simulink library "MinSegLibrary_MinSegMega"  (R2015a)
settings: Solver=ode45  StartTime=0.0  StopTime=10.0  RelTol=1e-3
undefined symbols (not defined in the file or in its folder): PWMoffset, Vsupply
libraries: MinSegLibrary_MinSegMega x7, MinSegLibrary_M1V4 x1

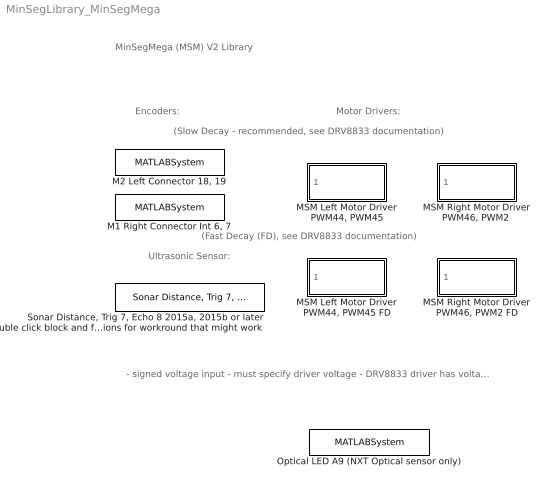
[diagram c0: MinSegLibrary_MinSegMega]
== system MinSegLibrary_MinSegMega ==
  note: (Slow Decay - recommended, see DRV8833 documentation)
  note: Motor Drivers:
  note: Ultrasonic Sensor:
  note: Encoders:
  note: MinSegMega (MSM) V2 Library
  note: (Fast Decay (FD), see DRV8833 documentation)
  note: - signed voltage input - must specify driver voltage - DRV8833 driver has voltage drop of about 0.6 volts, so max usable USB voltage is about 3.9 volts - Fast decay is nonlinear PWM to voltage for NXT motor - look at generic driver block in RASPlib for table lookup and other options
  "M1 Right Connector Int 6, 7" : MATLABSystem  System=Encoder_arduino  Encoder=2  PinA=6  PinB=7  PWMFSelect=3  PWMTimer=-1
  "M2 Left Connector 18, 19" : MATLABSystem  System=Encoder_arduino  Encoder=1  PinA=19  PinB=18  PWMFSelect=3  PWMTimer=-1
  "MSM Left Motor Driver PWM44, PWM45" : Subsystem
  "MSM Left Motor Driver PWM44, PWM45 FD" : Subsystem
  "MSM Right Motor Driver PWM46, PWM2 " : Subsystem
  "MSM Right Motor Driver PWM46, PWM2 FD" : Subsystem
  Optical LED A9 (NXT Optical sensor only) : MATLABSystem  System=soDAnalogWrite  Pin=9
  "Sonar Distance, Trig 7, Echo 8 2015a, 2015b or later double click block and follow instructions for workround that might work" : MinSegLibrary_M1V4/Sonar Distance, Trig 7, Echo 8 2015a, 2015b or later double click block and follow instructions for workround that might work  TrigPin=7  EchoPin=8

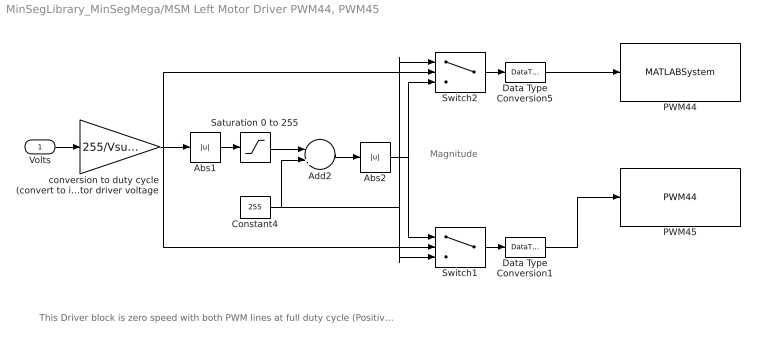
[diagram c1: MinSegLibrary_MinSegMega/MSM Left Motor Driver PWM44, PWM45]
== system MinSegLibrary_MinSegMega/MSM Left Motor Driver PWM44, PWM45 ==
  note: Magnitude
  note: This Driver block is zero speed with both PWM lines at full duty cycle (Positive voltage on both motor terminals). This method produces a linear motor response for DRV8833 driver in both directions and eliminates the typical dead zone when the motor starts. The driver may draw more current in this configuration (has not been verified) The SN754410 driver this has no effect, so the driver could alternatively be modified so that zero speed is zero voltage to both PWM lines.
  Volts : Inport
  Abs1 : Abs
  Abs2 : Abs
  Add2 : Sum  Inputs=-+
  Constant4 : Constant  Value=255
  Data Type Conversion1 : DataTypeConversion  OutDataTypeStr=uint8
  Data Type Conversion5 : DataTypeConversion  OutDataTypeStr=uint8
  PWM44 : MATLABSystem  System=soPWMWrite  Pin=44
  PWM45 : MinSegLibrary_MinSegMega/MSM Left Motor Driver PWM44, PWM45/PWM44  Pin=45
  Saturation 0 to 255 : Saturate  UpperLimit=255  LowerLimit=0
  Switch1 : Switch
  Switch2 : Switch
  conversion to duty cycle (convert to int) denominator is motor driver voltage : Gain  Gain=255/Vsupply  OutDataTypeStr=int16
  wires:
  Data Type Conversion1/1 -> PWM45/1
  Data Type Conversion5/1 -> PWM44/1
  Switch1/1 -> Data Type Conversion1/1
  Switch2/1 -> Data Type Conversion5/1
  Abs2/1 -> Switch1/1, Switch2/3
  Add2/1 -> Abs2/1
  Constant4/1 -> Add2/2, Switch2/1, Switch1/3
  Abs1/1 -> Saturation 0 to 255/1
  Saturation 0 to 255/1 -> Add2/1
  conversion to duty cycle (convert to int) denominator is motor driver voltage/1 -> Switch1/2, Abs1/1, Switch2/2
  Volts/1 -> conversion to duty cycle (convert to int) denominator is motor driver voltage/1

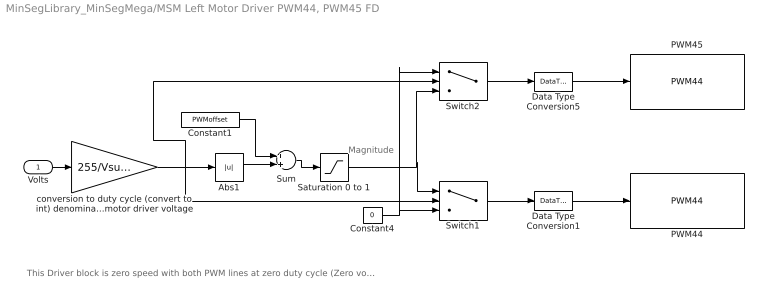
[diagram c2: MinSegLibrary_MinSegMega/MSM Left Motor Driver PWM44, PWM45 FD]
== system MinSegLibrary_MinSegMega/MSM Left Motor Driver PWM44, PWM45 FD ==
  note: Magnitude
  note: This Driver block is zero speed with both PWM lines at zero duty cycle (Zero voltage on both motor terminals). This method produces a nonlinear motor response for DRV8833 driver in both directions and eliminates
  Volts : Inport
  Abs1 : Abs
  Constant1 : Constant  Value=PWMoffset
  Constant4 : Constant  Value=0
  Data Type Conversion1 : DataTypeConversion  OutDataTypeStr=uint8
  Data Type Conversion5 : DataTypeConversion  OutDataTypeStr=uint8
  PWM44 : MinSegLibrary_MinSegMega/MSM Left Motor Driver PWM44, PWM45/PWM44  Pin=44
  PWM45 : MinSegLibrary_MinSegMega/MSM Left Motor Driver PWM44, PWM45/PWM44  Pin=45
  Saturation 0 to 1 : Saturate  UpperLimit=255  LowerLimit=0
  Sum : Sum
  Switch1 : Switch
  Switch2 : Switch
  conversion to duty cycle (convert to int) denominator is motor driver voltage : Gain  Gain=255/Vsupply  OutDataTypeStr=int16
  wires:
  Constant1/1 -> Sum/1
  Sum/1 -> Saturation 0 to 1/1
  Abs1/1 -> Sum/2
  Data Type Conversion1/1 -> PWM44/1
  Data Type Conversion5/1 -> PWM45/1
  Switch1/1 -> Data Type Conversion1/1
  Switch2/1 -> Data Type Conversion5/1
  Saturation 0 to 1/1 -> Switch1/1, Switch2/3
  Constant4/1 -> Switch1/3, Switch2/1
  conversion to duty cycle (convert to int) denominator is motor driver voltage/1 -> Switch2/2, Abs1/1, Switch1/2
  Volts/1 -> conversion to duty cycle (convert to int) denominator is motor driver voltage/1

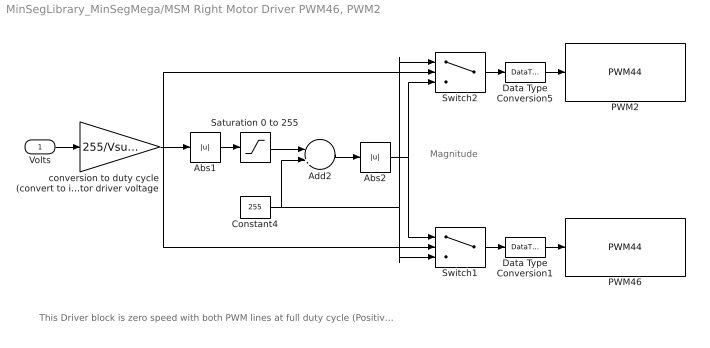
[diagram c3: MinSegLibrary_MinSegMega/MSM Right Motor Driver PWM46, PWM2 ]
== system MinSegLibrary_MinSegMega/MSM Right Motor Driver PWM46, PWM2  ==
  note: Magnitude
  note: This Driver block is zero speed with both PWM lines at full duty cycle (Positive voltage on both motor terminals). This method produces a linear motor response for DRV8833 driver in both directions and eliminates the typical dead zone when the motor starts. The driver may draw more current in this configuration (has not been verified) The SN754410 driver this has no effect, so the driver could alternatively be modified so that zero speed is zero voltage to both PWM lines.
  Volts : Inport
  Abs1 : Abs
  Abs2 : Abs
  Add2 : Sum  Inputs=-+
  Constant4 : Constant  Value=255
  Data Type Conversion1 : DataTypeConversion  OutDataTypeStr=uint8
  Data Type Conversion5 : DataTypeConversion  OutDataTypeStr=uint8
  PWM2 : MinSegLibrary_MinSegMega/MSM Left Motor Driver PWM44, PWM45/PWM44  Pin=2
  PWM46 : MinSegLibrary_MinSegMega/MSM Left Motor Driver PWM44, PWM45/PWM44  Pin=46
  Saturation 0 to 255 : Saturate  UpperLimit=255  LowerLimit=0
  Switch1 : Switch
  Switch2 : Switch
  conversion to duty cycle (convert to int) denominator is motor driver voltage : Gain  Gain=255/Vsupply  OutDataTypeStr=int16
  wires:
  Data Type Conversion1/1 -> PWM46/1
  Data Type Conversion5/1 -> PWM2/1
  Switch1/1 -> Data Type Conversion1/1
  Switch2/1 -> Data Type Conversion5/1
  Abs2/1 -> Switch1/1, Switch2/3
  Add2/1 -> Abs2/1
  Constant4/1 -> Add2/2, Switch2/1, Switch1/3
  Abs1/1 -> Saturation 0 to 255/1
  Saturation 0 to 255/1 -> Add2/1
  conversion to duty cycle (convert to int) denominator is motor driver voltage/1 -> Switch1/2, Switch2/2, Abs1/1
  Volts/1 -> conversion to duty cycle (convert to int) denominator is motor driver voltage/1

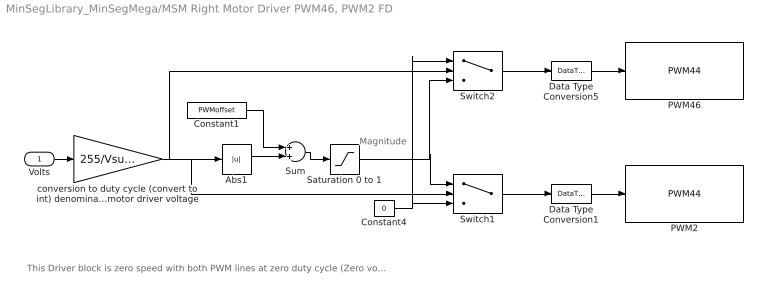
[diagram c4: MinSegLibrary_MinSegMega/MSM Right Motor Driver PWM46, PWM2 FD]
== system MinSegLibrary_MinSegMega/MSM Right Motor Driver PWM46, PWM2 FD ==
  note: Magnitude
  note: This Driver block is zero speed with both PWM lines at zero duty cycle (Zero voltage on both motor terminals). This method produces a nonlinear motor response for DRV8833 driver in both directions and eliminates
  Volts : Inport
  Abs1 : Abs
  Constant1 : Constant  Value=PWMoffset
  Constant4 : Constant  Value=0
  Data Type Conversion1 : DataTypeConversion  OutDataTypeStr=uint8
  Data Type Conversion5 : DataTypeConversion  OutDataTypeStr=uint8
  PWM2 : MinSegLibrary_MinSegMega/MSM Left Motor Driver PWM44, PWM45/PWM44  Pin=2
  PWM46 : MinSegLibrary_MinSegMega/MSM Left Motor Driver PWM44, PWM45/PWM44  Pin=46
  Saturation 0 to 1 : Saturate  UpperLimit=255  LowerLimit=0
  Sum : Sum
  Switch1 : Switch
  Switch2 : Switch
  conversion to duty cycle (convert to int) denominator is motor driver voltage : Gain  Gain=255/Vsupply  OutDataTypeStr=int16
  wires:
  Constant1/1 -> Sum/1
  Sum/1 -> Saturation 0 to 1/1
  Abs1/1 -> Sum/2
  Data Type Conversion1/1 -> PWM2/1
  Data Type Conversion5/1 -> PWM46/1
  Switch1/1 -> Data Type Conversion1/1
  Switch2/1 -> Data Type Conversion5/1
  Saturation 0 to 1/1 -> Switch1/1, Switch2/3
  Constant4/1 -> Switch1/3, Switch2/1
  conversion to duty cycle (convert to int) denominator is motor driver voltage/1 -> Switch2/2, Abs1/1, Switch1/2
  Volts/1 -> conversion to duty cycle (convert to int) denominator is motor driver voltage/1
